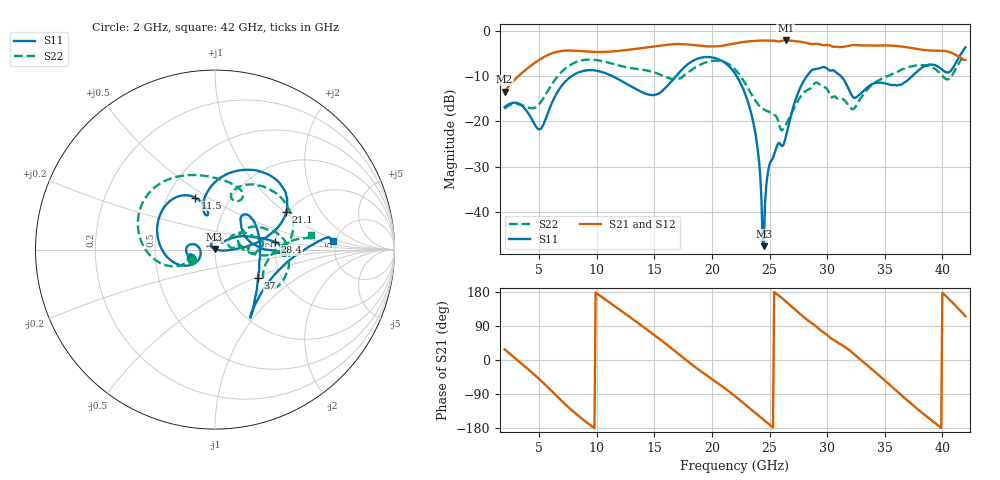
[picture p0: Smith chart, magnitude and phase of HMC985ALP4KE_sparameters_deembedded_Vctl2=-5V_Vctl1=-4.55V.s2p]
!s2p File: Measurements: S11, S21, S12, S22
# GHz S dB R 50.0
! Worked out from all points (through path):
!   401 points, 2 GHz to 42 GHz, reference 50 ohm
!   highest |S21| = -2.06 dB at 26.4 GHz (marker M1); lowest = -13.4 dB at 2 GHz (marker M2)
!   lowest |S11| = -47.6 dB at 24.5 GHz (marker M3), VSWR 1.01, Z = 49.7 + j0.311 ohm
!   |S11| at or under -10 dB: start of sweep to 7.806 GHz; 22.15 GHz to 28.23 GHz (6.083 GHz wide, 24.1 % of centre); 31.2 GHz to 37.36 GHz (6.157 GHz wide, 18 % of centre)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
!   |S22| runs from -21.9 to -5.3 dB; largest |S21 - S12| = 0.00079
!   S11 on the Smith chart (normalised r, x): 2 GHz: 0.76, -0.07; 11.5 GHz: 0.68, +0.44; 21.1 GHz: 1.97, +1.02; 28.4 GHz: 2.00, +0.19; 37 GHz: 1.52, -0.52; 42 GHz: 4.74, +0.84
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2  -16.87 -161.7  -13.43 28.2  -13.44 28.3  -17.17 -155.6
5  -21.78 -172.5  -6.38 -50.1  -6.38 -50.1  -16.18 -159.8
6.3  -14.83 -150.3  -4.76 -88.3  -4.76 -88.3  -11.03 -161.5
8.7  -8.90 150.4  -4.44 -154.5  -4.44 -154.5  -6.47 151.3
11.5  -10.15 111.1  -4.47 143.2  -4.47 143.2  -7.32 105.2
13.6  -13.11 101.2  -3.85 97.2  -3.85 97.2  -8.43 75.8
15.4  -13.81 105.8  -3.25 56.5  -3.25 56.5  -9.52 62.3
17.9  -7.33 80.3  -2.94 -3.5  -2.95 -3.4  -9.18 72.2
21.1  -6.98 27.6  -3.14 -74.3  -3.14 -74.3  -6.87 16.2
22  -9.38 17.0  -2.71 -95.5  -2.71 -95.5  -8.47 0.7
23.6  -20.35 -0.1  -2.18 -135.2  -2.18 -135.2  -14.73 -4.0
24.5  -47.65 131.1  -2.08 -157.9  -2.08 -157.8  -17.36 8.4
25  -29.46 133.3  -2.11 -170.6  -2.11 -170.6  -17.92 10.9
26.4  -23.55 42.4  -2.06 154.7  -2.06 154.8  -20.80 33.1
28.4  -9.42 7.2  -2.73 102.8  -2.73 102.8  -12.90 18.5
28.7  -8.61 2.2  -2.87 96.6  -2.87 96.6  -12.20 16.7
30.7  -8.96 -3.0  -3.45 50.8  -3.45 50.9  -14.48 2.5
32.5  -14.69 32.6  -3.09 10.9  -3.08 11.0  -16.61 28.2
35.4  -11.80 19.2  -3.18 -64.5  -3.18 -64.5  -9.81 19.5
37  -10.84 -33.3  -3.61 -107.6  -3.61 -107.6  -8.02 5.2
39.8  -8.16 -56.9  -4.32 -177.1  -4.31 -177.0  -9.33 -35.1
42  -3.60 4.3  -6.37 115.3  -6.38 115.4  -5.33 8.9
